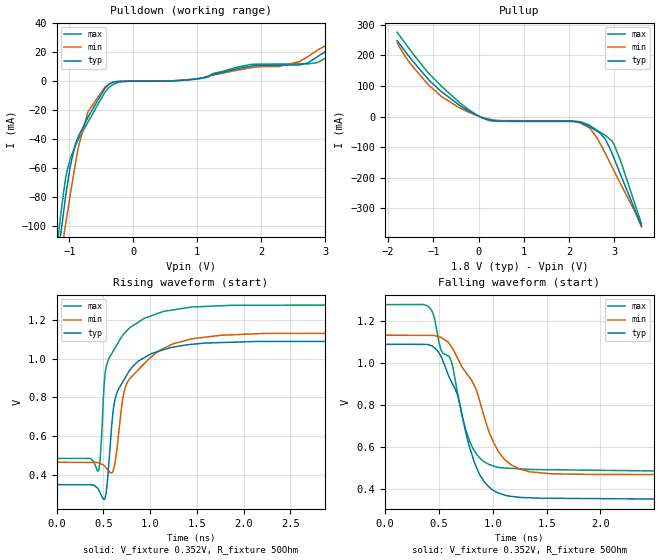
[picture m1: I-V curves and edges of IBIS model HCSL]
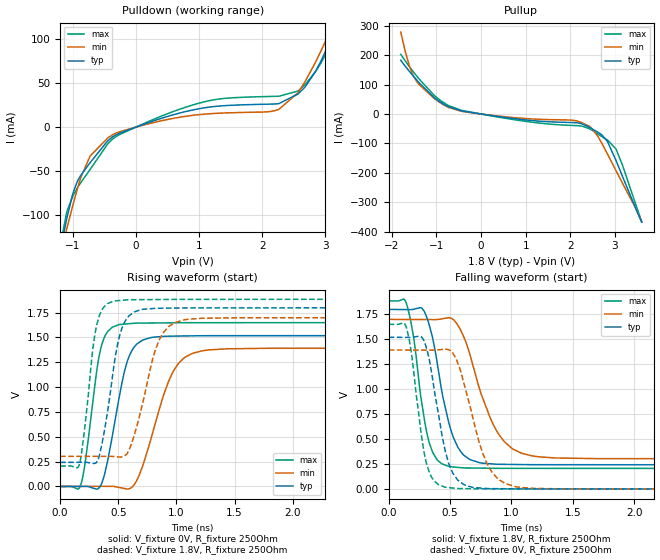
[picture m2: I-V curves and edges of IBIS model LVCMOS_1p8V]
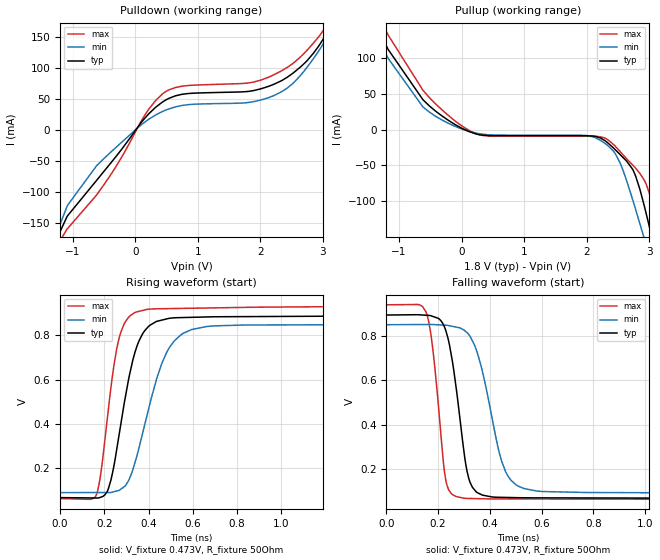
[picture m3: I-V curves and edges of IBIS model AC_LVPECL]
| Texas Instruments Incorporated
| Digital Temperature Sensor and Thermal Watchdog With Two-Wire Interface
| Marketing part#   Voltage Range   Package-type   #pins/pkg drawing
| LMK03328RHS   2.7V - 5.5V   WQFN   48-pin RHS
| LMK03318RHS   2.7V - 5.5V   WQFN   48-pin RHS
[IBIS Ver]   4.1
[File name]   lmk033x8.ibs
[File Rev]   1.3
[Date]   07/25/2017
[Source]   Model built from spectre simulations at:
   Texas Instruments Incorporated.
   Webench Design Center
   12500 TI Blvd
   Dallas, TX -75243
   For Support e-mail: elab_ibis@list.ti.com
[Notes]   Revision History
   Rev 1.3: 07/25/2017
   - Update HCSL model
   Rev 1.2: 10/08/2015
   - Correct pin assignnment on pins 16/17 and 23/24. Correct [Diff pin] statement as well
   Rev 1.1: 08/07/2015
   - Added OPEND and LVCMOS buffer models for STATUSn pins
   - LMK03318 component added
   Rev 1.0: 06/15/2015
   - Non monotonic behavior result of circuit behavior
   - ccomp values are based on PVT settings:
   MIN: Low Voltage, High Temperature, Weak Process
   TYP: Nominal Voltage, Nominal Temperature, Nominal Process
   MAX: High Voltage, Low Temperature, Fast Process
   - C_comp although listed in numerical order of value are obtained from varying PVT conditions.
   For PVT conditions for each specific value, refer to the buffer description under respective [Model].
   IBIS model user is responsible for using appropriate C_comp to simulate for Signal Integrity.
[Disclaimer]  This model is designed as an aid for customers of Texas Instruments
 TI and its licensors and suppliers make no warranties, either expressed
 or implied, with respect to this  model, including the warranties of
 merchantability or fitness for a particular purpose.
 The model is provided solely on an "as is" basis. The entire risk as to
 its quality and performance is with the customer.
[Copyright] (C)Copyright 2017 Texas Instruments Incorporated.
   All rights reserved.
[Component]   LMK03328RHS
[Manufacturer]  Texas Instruments Incorporated
[Package]   |48-pin WQFN RHS package
|   typ   min   max
R_pkg   0.261   0.138   0.370
L_pkg   1.288nH   0.780nH   1.750nH
C_pkg   45.2fF   34.6fF   106fF
[Pin]   signal_name   model_name   R_pin   L_pin   C_pin
1   STATUS0   STATUS   0.323   1.60n   4.65e-14
2   STATUS1   STATUS   0.298   1.43n   4.65e-14
3   CAP_DIG   NC   0.195   1.03n   4.55e-14
4   VCC_DIG   POWER   0.191   1.00n   5.31e-14
5   VDD_IN   POWER   0.176   0.97n   5.49e-14
6   PRIREF_P   NC   0.253   1.25n   5.49e-14
7   PRIREF_N   NC   0.234   1.18n   4.33e-14
8   REFSEL   NC   0.218   1.18n   3.87e-14
9   HW_SW_CTRL   NC   0.212   1.22n   4.36e-14
10   SECREF_P   NC   0.241   1.30n   4.58e-14
11   SECREF_N   NC   0.291   1.48n   4.58e-14
12   GPIO0   NC   0.326   1.59n   4.33e-14
13   PDN   NC   0.353   1.65n   4.24e-14
14   OUT0_P   MMD   0.345   1.59n   5.06e-14
15   OUT0_N   MMD   0.299   1.39n   5.06e-14
16   OUT1_N   MMD   0.294   1.37n   4.69e-14
17   OUT1_P   MMD   0.250   1.21n   4.69e-14
18   VDDO_01   POWER   0.141   0.80n   5.44e-14
19   VDDO_23   POWER   0.138   0.78n   5.44e-14
20   OUT2_P   MMD   0.230   1.14n   4.66e-14
21   OUT2_N   MMD   0.258   1.27n   4.66e-14
22   OUT3_N   MMD   0.277   1.31n   5.05e-14
23   OUT3_P   MMD   0.323   1.50n   5.03e-14
24   GPIO1   NC   0.343   1.60n   5.03e-14
25   SDA   NC   0.313   1.47n   4.65e-14
26   SCL   NC   0.278   1.32n   3.90e-14
27   VDD_PLL2   POWER   0.160   0.86n   3.91e-14
28   CAP_PLL2   NC   0.152   0.87n   3.91e-14
29   LF2   NC   0.248   1.22n   4.68e-14
30   GPIO2   NC   0.237   1.18n   4.68e-14
31   GPIO3   NC   0.243   1.19n   5.17e-14
32   GPIO4   NC   0.267   1.28n   5.55e-14
33   GPIO5   NC   0.309   1.49n   5.55e-14
34   LF1   NC   0.354   1.75n   4.82e-14
35   CAP_PLL1   NC   0.226   1.33n   4.54e-14
36   VDD_PLL1   POWER   0.205   1.16n   4.46e-14
37   VDD0_4   POWER   0.327   1.58n   4.88e-14
38   OUT4_N   MMD   0.304   1.42n   4.88e-14
39   OUT4_P   MMD   0.263   1.26n   3.62e-14
40   VDDO_5   POWER   0.263   1.27n   4.21e-14
41   OUT5_N   MMD   0.246   1.17n   4.21e-14
42   OUT5_P   MMD   0.226   1.12n   3.46e-14
43   VDDO_6   POWER   0.238   1.13n   4.40e-14
44   OUT6_N   MMD   0.239   1.14n   4.40e-14
45   OUT6_P   MMD   0.262   1.25n   4.00e-14
46   VDDO_7   POWER   0.270   1.33n   5.83e-14
47   OUT7_N   MMD   0.314   1.48n   1.06e-13
48   OUT7_P   MMD   0.370   1.71n   1.06e-13
[Diff pin]  inv_pin  vdiff  tdelay_typ  tdelay_min  tdelay_max
14   15   0.0   0.0s   0.0s   0.0s
17   16   0.0   0.0s   0.0s   0.0s
20   21   0.0   0.0s   0.0s   0.0s
23   22   0.0   0.0s   0.0s   0.0s
39   38   0.0   0.0s   0.0s   0.0s
42   41   0.0   0.0s   0.0s   0.0s
45   44   0.0   0.0s   0.0s   0.0s
48   47   0.0   0.0s   0.0s   0.0s
[Component]   LMK03318RHS
[Manufacturer]  Texas Instruments Incorporated
[Package]   |48-pin WQFN RHS package
|   typ   min   max
R_pkg   0.261   0.138   0.370
L_pkg   1.288nH   0.780nH   1.750nH
C_pkg   45.2fF   34.6fF   106fF
[Pin]   signal_name   model_name   R_pin   L_pin   C_pin
1   STATUS0   STATUS   0.323   1.60n   4.65e-14
2   STATUS1   STATUS   0.298   1.43n   4.65e-14
3   CAP_DIG   NC   0.195   1.03n   4.55e-14
4   VCC_DIG   POWER   0.191   1.00n   5.31e-14
5   VDD_IN   POWER   0.176   0.97n   5.49e-14
6   PRIREF_P   NC   0.253   1.25n   5.49e-14
7   PRIREF_N   NC   0.234   1.18n   4.33e-14
8   REFSEL   NC   0.218   1.18n   3.87e-14
9   HW_SW_CTRL   NC   0.212   1.22n   4.36e-14
10   SECREF_P   NC   0.241   1.30n   4.58e-14
11   SECREF_N   NC   0.291   1.48n   4.58e-14
12   GPIO0   NC   0.326   1.59n   4.33e-14
13   PDN   NC   0.353   1.65n   4.24e-14
14   OUT0_P   MMD   0.345   1.59n   5.06e-14
15   OUT0_N   MMD   0.299   1.39n   5.06e-14
16   OUT1_N   MMD   0.294   1.37n   4.69e-14
17   OUT1_P   MMD   0.250   1.21n   4.69e-14
18   VDDO_01   POWER   0.141   0.80n   5.44e-14
19   VDDO_23   POWER   0.138   0.78n   5.44e-14
20   OUT2_P   MMD   0.230   1.14n   4.66e-14
21   OUT2_N   MMD   0.258   1.27n   4.66e-14
22   OUT3_N   MMD   0.277   1.31n   5.05e-14
23   OUT3_P   MMD   0.323   1.50n   5.03e-14
24   GPIO1   NC   0.343   1.60n   5.03e-14
25   SDA   NC   0.313   1.47n   4.65e-14
26   SCL   NC   0.278   1.32n   3.90e-14
27   VDD_LDO   POWER   0.160   0.86n   3.91e-14
28   CAP_LDO   NC   0.152   0.87n   3.91e-14
29   NC   NC   0.248   1.22n   4.68e-14
30   GPIO2   NC   0.237   1.18n   4.68e-14
31   GPIO3   NC   0.243   1.19n   5.17e-14
32   GPIO4   NC   0.267   1.28n   5.55e-14
33   GPIO5   NC   0.309   1.49n   5.55e-14
34   LF   NC   0.354   1.75n   4.82e-14
35   CAP_PLL   NC   0.226   1.33n   4.54e-14
36   VDD_PLL   POWER   0.205   1.16n   4.46e-14
37   VDD0_4   POWER   0.327   1.58n   4.88e-14
38   OUT4_N   MMD   0.304   1.42n   4.88e-14
39   OUT4_P   MMD   0.263   1.26n   3.62e-14
40   VDDO_5   POWER   0.263   1.27n   4.21e-14
41   OUT5_N   MMD   0.246   1.17n   4.21e-14
42   OUT5_P   MMD   0.226   1.12n   3.46e-14
43   VDDO_6   POWER   0.238   1.13n   4.40e-14
44   OUT6_N   MMD   0.239   1.14n   4.40e-14
45   OUT6_P   MMD   0.262   1.25n   4.00e-14
46   VDDO_7   POWER   0.270   1.33n   5.83e-14
47   OUT7_N   MMD   0.314   1.48n   1.06e-13
48   OUT7_P   MMD   0.370   1.71n   1.06e-13
[Diff pin]  inv_pin  vdiff  tdelay_typ  tdelay_min  tdelay_max
14   15   0.0   0.0s   0.0s   0.0s
17   16   0.0   0.0s   0.0s   0.0s
20   21   0.0   0.0s   0.0s   0.0s
23   22   0.0   0.0s   0.0s   0.0s
39   38   0.0   0.0s   0.0s   0.0s
42   41   0.0   0.0s   0.0s   0.0s
45   44   0.0   0.0s   0.0s   0.0s
48   47   0.0   0.0s   0.0s   0.0s
[Model Selector] STATUS
OPEND_3p3V_fast   3.3V Open Drain, Fast Tr/Tf
OPEND_3p3V_slow   3.3V Open Drain, Slow Tr/Tf
LVCMOS_3p3V_fast   3.3V CMOS, Fast Tr/Tf
LVCMOS_3p3V_slow   3.3V CMOS, slow Tr/Tf
[Model Selector] MMD
HCSL   1.8V HCSL
LVCMOS_1p8V  1.8V LVCMOS
AC_LVPECL   1.8V LVPECL
AC_CML   1.8V CML
AC_LVDS   1.8V LVDS
| Models and submodels in the file (9): HCSL (Output), LVCMOS_1p8V (Output), AC_LVPECL (Output), AC_LVDS (Output), AC_CML (Output), OPEND_3p3V_slow (Open_drain), OPEND_3p3V_fast (Open_drain), LVCMOS_3p3V_slow (3-state), LVCMOS_3p3V_fast (3-state)
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|   Model IN_3P3V
[Model]   HCSL
Model_type   Output
Polarity   Non-Inverting
Vmeas = 0.4
Vref = 0.0
Cref = 2pF
Rref = 50
|   typ   min   max
|   (nom PVT)   (fast PVT)   (slow PVT)
C_comp   0.989p   0.973p   0.998p
|C_comp (ON state)   0.989p   0.973p   0.998p
|C_comp (OFF state)   0.989p   0.973p   0.998p
| Where   nom PVT is  Nominal Process, 1.8V, 27C
|   Fast PVT is Strong Process, 1.9V, -40C
|   Slow PVT is Weak Process, 1.7V, 125C
[Voltage Range]   1.8   1.7   1.9
[Temperature Range]   27   125   -40
[Pullup Reference]   1.8   1.7   1.9
[Pulldown Reference]   0   0   0
[Power Clamp Reference]   1.8   1.7   1.9
[GND Clamp Reference]   0   0   0
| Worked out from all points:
|   slope of the pullup table from 0 to 0.27 V, typ, clamps not added: 20.3 ohm
|   falling waveform, V_fixture 0.352V, R_fixture 50Ohm: 20-80 % time 264ps typ, 334ps min, 280ps max; typ from 1.09 V to 0.352 V
|   rising waveform, V_fixture 0.352V, R_fixture 50Ohm: 20-80 % time 220ps typ, 326ps min, 223ps max; typ from 0.352 V to 1.09 V
[Pulldown]
|   Voltage   I(typ)   I(min)   I(max)
-1.8V     -347.1mA   -316.3mA   -384.6mA
-1.211V   -133.8mA   -144.1mA   -123.6mA
-1.136V   -106.3mA   -121.8mA   -92.64mA
-1.066V   -82.3mA    -101.2mA   -69.03mA
-903.6mV  -43.28mA   -56.53mA   -44.41mA
-709.2mV  -24.91mA   -21.11mA   -28.31mA
-358.2mV  -1.553mA   -1.373mA   -3.551mA
2.876V    16.97mA    21.49mA    12.91mA
3.071V    27.66mA    29.42mA    26.35mA
3.092V    27.98mA    21.33mA    28.01mA
3.109V    17.68mA    21.81mA    12.65mA
3.6V      35.09mA    36.44mA    32.61mA
[Pullup]
|   Voltage   I(typ)   I(min)   I(max)
-1.8V     249mA      242.1mA    275.8mA
-1.465V   183.5mA    165.3mA    208.4mA
-817.2mV  81.16mA    65.18mA    98.7mA
57.6mV    -2.052mA   -1.327mA   -2.634mA
370.8mV   -13.84mA   -11.68mA   -15.3mA
2.115V    -15.32mA   -16.03mA   -16.02mA
2.466V    -34.62mA   -39.71mA   -30.19mA
2.671V    -52.84mA   -84.28mA   -49.99mA
2.806V    -75.45mA   -122.6mA   -62.33mA
2.995V    -137.3mA   -178.4mA   -91.86mA
3.141V    -191.4mA   -221.2mA   -146.4mA
3.6V      -356.9mA   -361.9mA   -351mA
[Ramp]
R_load = 50
|   typ   min   max
dV/dt_r   0.441924/2.19244e-10   0.398252/3.25048e-10   0.474499/2.21894e-10
dV/dt_f   0.194/2.62871e-10   0.159/3.34277e-10   0.2312/2.79025e-10
[Falling Waveform]
V_fixture = 0.352V
V_fixture_min = 0.467V
V_fixture_max = 0.487V
R_fixture = 50Ohm
C_fixture = 0F
|   Time   V(typ)   V(min)   V(max)
0s        1.088V     1.131V     1.277V
396.8ps   1.088V     1.131V     1.271V
493.5ps   1.053V     1.125V     1.12V
617.5ps   909.9mV    1.076V     1.005V
721.2ps   738.6mV    975.2mV    737.9mV
802.9ps   571mV      918.5mV    608.1mV
1.025ns   389mV      605.2mV    507.3mV
1.247ns   361.7mV    496.4mV    497.1mV
1.545ns   357.3mV    473.5mV    492.8mV
7ns       352.3mV    466.8mV    488mV
[Rising Waveform]
V_fixture = 0.352V
V_fixture_min = 0.467V
V_fixture_max = 0.487V
R_fixture = 50Ohm
C_fixture = 0F
|   Time   V(typ)   V(min)   V(max)
0s        352mV      467.1mV    487mV
448.3ps   328mV      464.7mV    422.4mV
468.1ps   308.4mV    460.4mV    491.6mV
513.7ps   276.4mV    446.9mV    892.3mV
599.2ps   701.9mV    417mV      1.033V
653.7ps   834mV      566.9mV    1.077V
751.7ps   915.4mV    872.1mV    1.143V
1.144ns   1.045V     1.052V     1.242V
2.244ns   1.088V     1.129V     1.274V
7ns       1.089V     1.131V     1.278V
[Model]   LVCMOS_1p8V
Model_type   Output
Polarity   Non-Inverting
Vmeas = 0.9
Vref = 1.8
Cref = 15pF
Rref = 250
|   typ   min   max
|   (nom PVT)   (fast PVT)   (slow PVT)
C_comp   0.989p   0.973p   0.998p
|C_comp (ON state)   0.989p   0.973p   0.998p
|C_comp (OFF state)   0.989p   0.973p   0.998p
| Where   nom PVT is  Nominal Process, 1.8V, 27C
|   Fast PVT is Strong Process, 1.9V, -40C
|   Slow PVT is Weak Process, 1.7V, 125C
[Voltage Range]   1.8   1.7   1.9
[Temperature Range]   27   125   -40
[Pullup Reference]   1.8   1.7   1.9
[Pulldown Reference]   0   0   0
[Power Clamp Reference]   1.8   1.7   1.9
[GND Clamp Reference]   0   0   0
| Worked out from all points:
|   slope of the pulldown table from 0 to 0.27 V, typ, clamps not added: 39.1 ohm
|   slope of the pullup table from 0 to 0.27 V, typ, clamps not added: 43.7 ohm
|   falling waveform, V_fixture 1.8V, R_fixture 250Ohm: 20-80 % time 155ps typ, 237ps min, 116ps max; typ from 1.8 V to 0.242 V
|   rising waveform, V_fixture 0V, R_fixture 250Ohm: 20-80 % time 151ps typ, 225ps min, 111ps max; typ from 0 V to 1.52 V
|   rising waveform, V_fixture 1.8V, R_fixture 250Ohm: 20-80 % time 126ps typ, 180ps min, 95.4ps max; typ from 0.242 V to 1.8 V
|   falling waveform, V_fixture 0V, R_fixture 250Ohm: 20-80 % time 135ps typ, 192ps min, 104ps max; typ from 1.52 V to 0 V
[Pulldown]
|   Voltage   I(typ)   I(min)   I(max)
-1.8V     -353.1mA   -318.4mA   -395.7mA
-1.238V   -154.2mA   -156.3mA   -149.5mA
-1.093V   -103.1mA   -114.8mA   -95.95mA
-930.6mV  -62.18mA   -71.08mA   -69.5mA
-725.4mV  -40.34mA   -32.92mA   -48.13mA
-369mV    -11.06mA   -8.672mA   -13.55mA
1.067V    21.77mA    14.67mA    28.53mA
2.266V    26.75mA    20.29mA    35.15mA
2.682V    45.79mA    51.94mA    48.47mA
2.936V    75.68mA    87.11mA    73.28mA
3.163V    113mA      126mA      107.6mA
3.6V      199.5mA    353.2mA    196.6mA
[Pullup]
|   Voltage   I(typ)   I(min)   I(max)
-1.8V     182.8mA    278.7mA    202.8mA
-1.606V   145mA      163.3mA    161.2mA
-1.433V   113.9mA    108.4mA    127.3mA
-1.055V   56.58mA    53.59mA    64.17mA
-768.6mV  27.58mA    25.08mA    31.94mA
613.8mV   -13.34mA   -10.49mA   -16.24mA
2.131V    -29.75mA   -23.31mA   -39.51mA
2.466V    -48.61mA   -46.2mA    -53.06mA
2.698V    -69.78mA   -97.28mA   -76.04mA
2.844V    -97.34mA   -139.3mA   -89.96mA
3.028V    -159.5mA   -193.7mA   -120.3mA
3.6V      -368mA     -366.8mA   -366.7mA
[Ramp]
R_load = 250
|   typ   min   max
dV/dt_r   0.912017/1.49886e-10   0.836011/2.23854e-10   0.990371/1.10706e-10
dV/dt_f   0.934331/1.54327e-10   0.838292/2.3661e-10   1.00765/1.15451e-10
[Falling Waveform]
V_fixture = 1.8V
V_fixture_min = 1.7V
V_fixture_max = 1.9V
R_fixture = 250Ohm
C_fixture = 0F
|   Time   V(typ)   V(min)   V(max)
0s        1.799V     1.7V       1.885V
151ps     1.798V     1.699V     1.834V
203.2ps   1.801V     1.698V     1.518V
289.4ps   1.78V      1.698V     709.1mV
359.1ps   1.506V     1.698V     365.9mV
493.1ps   651.4mV    1.716V     226.6mV
614.6ps   337.1mV    1.515V     212.3mV
886.9ps   249.1mV    568.1mV    208.8mV
1.165ns   245.2mV    333.7mV    208.3mV
6.3ns     242.1mV    302.4mV    205.7mV
[Rising Waveform]
V_fixture = 0V
V_fixture_min = 0V
V_fixture_max = 0V
R_fixture = 250Ohm
C_fixture = 0F
|   Time   V(typ)   V(min)   V(max)
0s        -12.06uV   5.904uV    -65.22uV
180ps     843.2uV    552.6uV    25.69mV
345.6ps   1.689mV    1.056mV    1.369V
403.4ps   232.2mV    1.231mV    1.55V
505.6ps   884mV      -9.912mV   1.628V
576.7ps   1.257V     -26.07mV   1.636V
661.6ps   1.435V     67.2mV     1.643V
966.4ps   1.512V     1.145V     1.646V
1.219ns   1.516V     1.364V     1.647V
6.3ns     1.52V      1.393V     1.651V
[Rising Waveform]
V_fixture = 1.8V
V_fixture_min = 1.7V
V_fixture_max = 1.9V
R_fixture = 250Ohm
C_fixture = 0F
|   Time   V(typ)   V(min)   V(max)
0s        242.1mV    302.4mV    205.5mV
167.5ps   242.8mV    302.6mV    229.9mV
279.6ps   233.1mV    302.8mV    1.372V
321.3ps   256.3mV    302.8mV    1.655V
460.7ps   1.202V     301.2mV    1.865V
517.4ps   1.543V     295.5mV    1.871V
591.9ps   1.717V     365.5mV    1.878V
842ps     1.793V     1.447V     1.88V
1.063ns   1.795V     1.675V     1.882V
6.3ns     1.799V     1.7V       1.885V
[Falling Waveform]
|Gnd
V_fixture = 0V
V_fixture_min = 0V
V_fixture_max = 0V
R_fixture = 250Ohm
C_fixture = 0F
|   Time   V(typ)   V(min)   V(max)
0s        1.52V      1.393V     1.65V
147.5ps   1.519V     1.393V     1.603V
187.1ps   1.519V     1.393V     1.347V
285.4ps   1.491V     1.392V     388.9mV
348.6ps   1.173V     1.392V     121.7mV
461.5ps   377.5mV    1.401V     18.99mV
580.9ps   74.02mV    1.203V     5.796mV
808.3ps   5.882mV    237.1mV    3.25mV
1.031ns   3.09mV     25.37mV    2.539mV
6.3ns     116.3uV    5.904uV    46.54uV
[Model]   AC_LVPECL
Model_type   Output
Polarity   Non-Inverting
Vmeas = 0.4
Vref = 0.473
Cref = 15pF
Rref = 50
|   typ   min   max
|   (nom PVT)   (fast PVT)   (slow PVT)
C_comp   0.989p   0.973p   0.998p
|C_comp (ON state)   0.989p   0.973p   0.998p
|C_comp (OFF state)   0.989p   0.973p   0.998p
| Where   nom PVT is  Nominal Process, 1.8V, 27C
|   Fast PVT is Strong Process, 1.9V, -40C
|   Slow PVT is Weak Process, 1.7V, 125C
[Voltage Range]   1.8   1.7   1.9
[Temperature Range]   27   125   -40
[Pullup Reference]   1.8   1.7   1.9
[Pulldown Reference]   0   0   0
[Power Clamp Reference]   1.8   1.7   1.9
[GND Clamp Reference]   0   0   0
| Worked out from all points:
|   slope of the pulldown table from 0 to 0.27 V, typ, clamps not added: 8.34 ohm
|   slope of the pullup table from 0 to 0.27 V, typ, clamps not added: 30.4 ohm
|   falling waveform, V_fixture 0.473V, R_fixture 50Ohm: 20-80 % time 56.7ps typ, 86.1ps min, 42.8ps max; typ from 0.892 V to 0.069 V
|   rising waveform, V_fixture 0.473V, R_fixture 50Ohm: 20-80 % time 92.7ps typ, 127ps min, 69.2ps max; typ from 0.069 V to 0.892 V
[Pulldown]
|   Voltage   I(typ)   I(min)   I(max)
-2.5V     -644mA     -811mA     -652.9mA
-1.315V   -189.5mA   -182.4mA   -198.6mA
-1.09V    -140.3mA   -123.9mA   -160.6mA
-512.5mV  -68.72mA   -47.73mA   -90.53mA
222.5mV   26.4mA     17.38mA    34.07mA
537.5mV   50.7mA     33.69mA    64.39mA
1.798V    61.85mA    43.92mA    75.48mA
2.217V    73.57mA    55.3mA     88.92mA
2.638V    101.2mA    87.39mA    117.4mA
3.058V    155.1mA    147.6mA    167.9mA
3.147V    170.4mA    163.9mA    182.5mA
5V        948.9mA    1.026A     845.1mA
[Pullup]
|   Voltage   I(typ)   I(min)   I(max)
-2.5V     561.1mA    647.4mA    493.8mA
-1.6V     192.7mA    186mA      218.7mA
-1.195V   116.1mA    103.3mA    136.4mA
-617.5mV  42.07mA    31.97mA    55.35mA
245mV     -6.127mA   -4.866mA   -5.995mA
2.225V    -11.79mA   -15.15mA   -9.974mA
2.533V    -34.55mA   -46.09mA   -30.27mA
2.743V    -56.64mA   -100mA     -50.03mA
2.915V    -104.7mA   -150.6mA   -69.75mA
3.005V    -136.8mA   -177.2mA   -89.85mA
3.147V    -189.8mA   -219mA     -145.3mA
5V        -1.262A    -1.547A    -1.056A
[Ramp]
R_load = 50
|   typ   min   max
dV/dt_r   0.494089/9.26499e-11   0.454514/1.26495e-10   0.524219/6.91641e-11
dV/dt_f   0.494089/5.64959e-11   0.454514/8.57846e-11   0.524219/4.2745e-11
[Falling Waveform]
V_fixture = 0.473V
V_fixture_min = 0.467V
V_fixture_max = 0.487V
R_fixture = 50Ohm
C_fixture = 0F
|   Time   V(typ)   V(min)   V(max)
0s        892mV      848.6mV    938mV
152.4ps   891.1mV    849.5mV    907.4mV
182ps     884.7mV    849.2mV    712.4mV
230.1ps   820.9mV    846.3mV    147.4mV
258.1ps   661.8mV    840.6mV    83.76mV
296.7ps   307.3mV    826.8mV    69.66mV
332.5ps   118.2mV    775.8mV    67.63mV
460.4ps   72.57mV    189.8mV    65.78mV
580.9ps   70.73mV    101.5mV    65.59mV
6.7ns     68.52mV    91.04mV    64.29mV
[Rising Waveform]
V_fixture = 0.473V
V_fixture_min = 0.467V
V_fixture_max = 0.487V
R_fixture = 50Ohm
C_fixture = 0F
|   Time   V(typ)   V(min)   V(max)
0s        68.52mV    91.04mV    64.29mV
159ps     66.96mV    91.33mV    72.24mV
182ps     69.82mV    91.37mV    164.9mV
211.4ps   93.27mV    91.43mV    407.1mV
273.6ps   394.2mV    105.9mV    810.4mV
329.9ps   692.1mV    197.9mV    896.4mV
392ps     830.7mV    434.8mV    915.8mV
515.5ps   878mV      773.3mV    919.8mV
698.2ps   882.8mV    841.8mV    922.8mV
6.7ns     892mV      848.6mV    938mV
